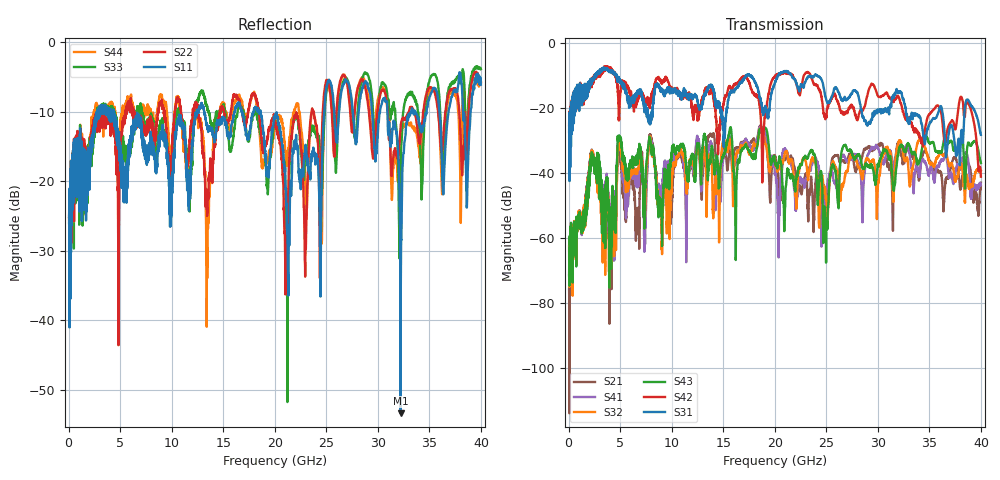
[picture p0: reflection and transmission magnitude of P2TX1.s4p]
!Agilent Technologies,N5245A,MY49151084,A.09.20.08
!Agilent N5245A: A.09.20.08
!Date: Thursday, March 01, 2012 13:15:54
!Correction: S11(Full 4 Port(1,2,3,4))
!S12(Full 4 Port(1,2,3,4))
!S13(Full 4 Port(1,2,3,4))
!S14(Full 4 Port(1,2,3,4))
!S21(Full 4 Port(1,2,3,4))
!S22(Full 4 Port(1,2,3,4))
!S23(Full 4 Port(1,2,3,4))
!S24(Full 4 Port(1,2,3,4))
!S31(Full 4 Port(1,2,3,4))
!S32(Full 4 Port(1,2,3,4))
!S33(Full 4 Port(1,2,3,4))
!S34(Full 4 Port(1,2,3,4))
!S41(Full 4 Port(1,2,3,4))
!S42(Full 4 Port(1,2,3,4))
!S43(Full 4 Port(1,2,3,4))
!S44(Full 4 Port(1,2,3,4))
!S4P File: Measurements: <S11,S12,S13,S14>,
!<S21,S22,S23,S24>,
!<S31,S32,S33,S34>,
!<S41,S42,S43,S44>:
# Hz S  dB  R 50
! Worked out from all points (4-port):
!   3996 points, 50 MHz to 40 GHz, reference 50 ohm
!   strongest paths, dB at 50 MHz, 10.04 GHz, 20.03 GHz, 30.02 GHz, 40 GHz:
!     S31: -27.4, -14.1, -11.9, -20.9, -28.2
!     S42: -25.3, -14.3, -10.1, -16.3, -41.1
!     S43: -71.5, -32.0, -36.8, -37.8, -36.9
!     S32: -62.5, -39.9, -36.3, -42.7, -39.1
!     S41: -70.9, -37.4, -40.4, -32.1, -43.7
!     S21: -75.8, -46.5, -35.1, -31.3, -42.9
!   lowest |S11| = -53.4 dB at 32.21 GHz (marker M1), VSWR 1.00, Z = 49.8 - j0.127 ohm
!   |S11| at or under -10 dB: 4.362 GHz to 12.48 GHz (8.119 GHz wide, 96.4 % of centre); 13.15 GHz to 16.11 GHz (2.957 GHz wide, 20.2 % of centre); 18.63 GHz to 24.79 GHz (6.166 GHz wide, 28.4 % of centre)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
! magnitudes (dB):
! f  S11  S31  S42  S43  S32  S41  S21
! 50 MHz  -25.1  -27.4  -25.3  -71.5  -62.5  -70.9  -75.8
! 2.27 GHz  -13.3  -11.6  -12.5  -35.4  -34.3  -35.8  -34.4
! 8.9 GHz  -13.5  -13.8  -11.5  -50.6  -49.9  -45.0  -47.0
! 19.01 GHz  -14.2  -20.6  -23.1  -26.2  -29.7  -26.9  -29.2
! 24.87 GHz  -8.4  -16.1  -22.6  -54.0  -44.6  -54.0  -50.1
! 32.21 GHz  -53.4  -15.0  -18.5  -31.9  -30.3  -31.9  -33.5
! 40 GHz  -6.1  -28.2  -41.1  -36.9  -39.1  -43.7  -42.9
